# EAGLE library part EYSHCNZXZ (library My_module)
Wireless Module: Bluetooth Smart (BLE)
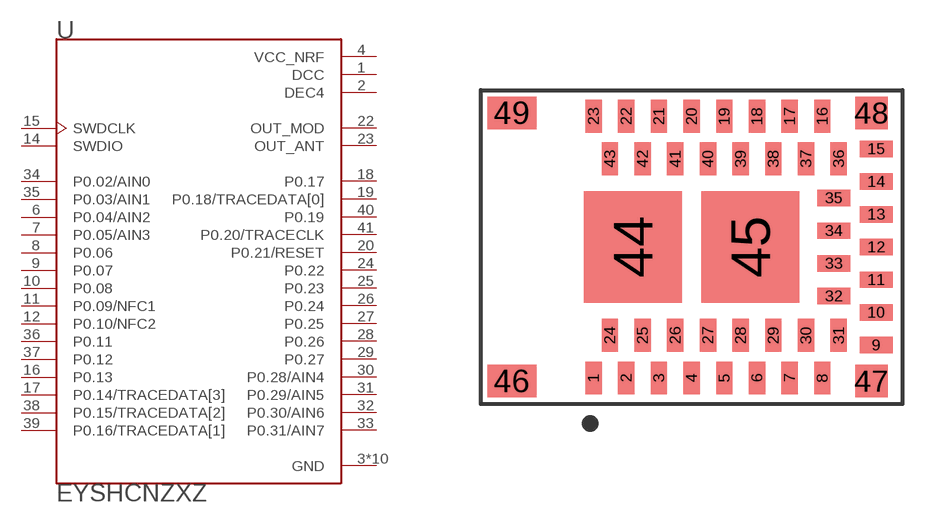
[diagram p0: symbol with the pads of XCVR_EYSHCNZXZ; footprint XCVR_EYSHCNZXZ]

Designator prefix U

## EYSHCNZXZ (DESCRIPTION: Wireless Module: Bluetooth? Smart _BLE_; MP: EYSHCNZXZ)  [XCVR_EYSHCNZXZ]
1  DCC  pwr
2  DEC4  pwr
3  GND  pwr
4  VCC_NRF  pwr
5  GND  pwr
6  P0.04/AIN2
7  P0.05/AIN3
8  P0.06
9  P0.07
10  P0.08
11  P0.09/NFC1
12  P0.10/NFC2
13  GND  pwr
14  SWDIO
15  SWDCLK  in
16  P0.13
17  P0.14/TRACEDATA[3]
18  P0.17
19  P0.18/TRACEDATA[0]
20  P0.21/RESET
21  GND  pwr
22  OUT_MOD
23  OUT_ANT
24  P0.22
25  P0.23
26  P0.24
27  P0.25
28  P0.26
29  P0.27
30  P0.28/AIN4
31  P0.29/AIN5
32  P0.30/AIN6
33  P0.31/AIN7
34  P0.02/AIN0
35  P0.03/AIN1
36  P0.11
37  P0.12
38  P0.15/TRACEDATA[2]
39  P0.16/TRACEDATA[1]
40  P0.19
41  P0.20/TRACECLK
42  GND  pwr
43  GND  pwr
44  GND  pwr
45  GND  pwr
47  GND  pwr
48  GND  pwr

## EYSHCNZXZNEW  [XCVR_EYSHCNZXZ]

## Footprint XCVR_EYSHCNZXZ (pad centres in mm)
smd 0.5 x 1: 1 -3,-4; 2 -2,-4; 3 -1,-4; 4 0,-4; 5 1,-4; 6 2,-4; 7 3,-4; 8 4,-4; 16 4,4; 17 3,4; 18 2,4; 19 1,4; 20 0,4; 21 -1,4; 22 -2,4; 23 -3,4; 24 -2.5,-2.7; 25 -1.5,-2.7; 26 -0.5,-2.7; 27 0.5,-2.7; 28 1.5,-2.7; 29 2.5,-2.7; 30 3.5,-2.7; 31 4.5,-2.7; 36 4.5,2.7; 37 3.5,2.7; 38 2.5,2.7; 39 1.5,2.7; 40 0.5,2.7; 41 -0.5,2.7; 42 -1.5,2.7; 43 -2.5,2.7
smd 1 x 0.5: 9 5.65,-3; 10 5.65,-2; 11 5.65,-1; 12 5.65,0; 13 5.65,1; 14 5.65,2; 15 5.65,3; 32 4.35,-1.5; 33 4.35,-0.5; 34 4.35,0.5; 35 4.35,1.5
smd 3 x 3.4: 44 -1.8,0; 45 1.8,0
smd 1.5 x 1: 46 -5.5,-4.1; 49 -5.5,4.1
smd 1 x 1: 47 5.5,-4.1; 48 5.5,4.1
